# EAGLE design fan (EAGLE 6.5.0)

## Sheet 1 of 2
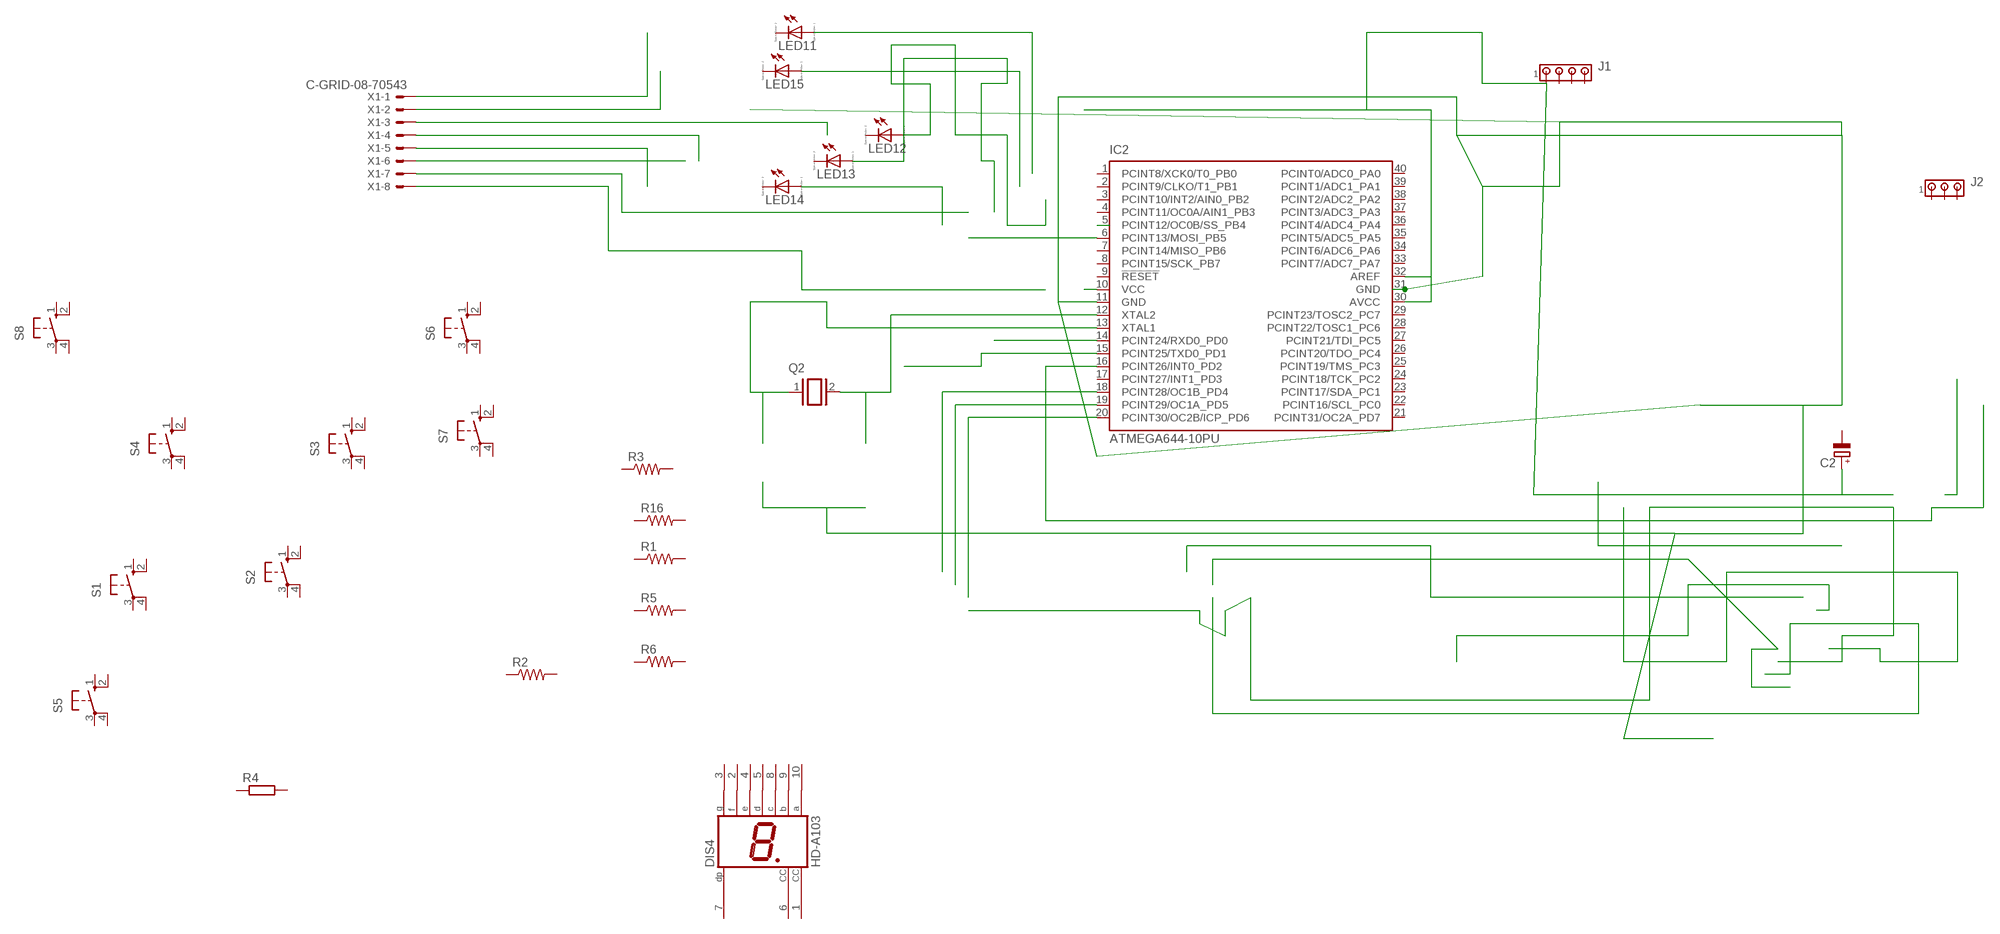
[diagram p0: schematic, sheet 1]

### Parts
C2  CPOL-EUE2,5-6E  [E2,5-6E]
DIS4  HD-A103  [HDSP-A]
IC2  ATMEGA644-10PU  [DIL40]
J1  MTA04-100  [10X04MTA]
J2  MTA03-100  [10X03MTA]
LED11  LED_ELD260  [LED_LD260]
LED12  LED_ELD260  [LED_LD260]
LED13  LED_ELD260  [LED_LD260]
LED14  LED_ELD260  [LED_LD260]
LED15  LED_ELD260  [LED_LD260]
Q2  XTAL/S  [QS]
R1  R-US_0204/2V  [0204V]
R2  R-US_0204/7  [0204/7]
R3  R-US_0204/7  [0204/7]
R4  R-EU_0207/2V  [0207/2V]
R5  R-US_0204/7  [0204/7]
R6  R-US_0204/7  [0204/7]
R16  R-US_0204/7  [0204/7]
S1  10-XX  [B3F-10XX]
S2  10-XX  [B3F-10XX]
S3  10-XX  [B3F-10XX]
S4  10-XX  [B3F-10XX]
S5  10-XX  [B3F-10XX]
S6  10-XX  [B3F-10XX]
S7  10-XX  [B3F-10XX]
S8  10-XX  [B3F-10XX]
X1  C-GRID-08-70543  [70543-08]

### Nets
N$2: IC2.13(XTAL1) Q2.1
N$3: IC2.16(PCINT26/INT0_PD2)
N$4: IC2.12(XTAL2) Q2.2
N$5: LED15.A
N$6: IC2.6(PCINT13/MOSI_PB5)
N$7: C2.+ IC2.30(AVCC) IC2.32(AREF) J1.1
N$9: LED14.A
N$11: X1.1
N$12: LED13.A
N$13: LED12.A
N$14: IC2.18(PCINT28/OC1B_PD4)
N$15: IC2.19(PCINT29/OC1A_PD5)
N$16: IC2.20(PCINT30/OC2B/ICP_PD6)
N$18: IC2.15(PCINT25/TXD0_PD1)
N$22: X1.2
N$24: X1.8
N$30: LED11.A
N$31: IC2.14(PCINT24/RXD0_PD0)
N$36: X1.4
N$37: X1.5
N$38: X1.7
N$39: X1.3
N$40: X1.6
N$43: IC2.11(GND) IC2.31(GND)
N$56: IC2.5(PCINT12/OC0B/SS_PB4)
N$66: IC2.10(VCC)
Unconnected: C2.- DIS4.1(CC) DIS4.2(F) DIS4.3(G) DIS4.4(E) DIS4.5(D) DIS4.6(CC) DIS4.7(DP) DIS4.8(C) DIS4.9(B) DIS4.10(A) IC2.1(PCINT8/XCK0/T0_PB0) IC2.2(PCINT9/CLKO/T1_PB1) IC2.3(PCINT10/INT2/AIN0_PB2) IC2.4(PCINT11/OC0A/AIN1_PB3) IC2.7(PCINT14/MISO_PB6) IC2.8(PCINT15/SCK_PB7) IC2.9(!RESET) IC2.17(PCINT27/INT1_PD3) IC2.21(PCINT31/OC2A_PD7) IC2.22(PCINT16/SCL_PC0) IC2.23(PCINT17/SDA_PC1) IC2.24(PCINT18/TCK_PC2) IC2.25(PCINT19/TMS_PC3) IC2.26(PCINT20/TDO_PC4) IC2.27(PCINT21/TDI_PC5) IC2.28(PCINT22/TOSC1_PC6) IC2.29(PCINT23/TOSC2_PC7) IC2.33(PCINT7/ADC7_PA7) IC2.34(PCINT6/ADC6_PA6) IC2.35(PCINT5/ADC5_PA5) IC2.36(PCINT4/ADC4_PA4) IC2.37(PCINT3/ADC3_PA3) IC2.38(PCINT2/ADC2_PA2) IC2.39(PCINT1/ADC1_PA1) IC2.40(PCINT0/ADC0_PA0) J1.2 J1.3 J1.4 J2.1 J2.2 J2.3 LED11.K(C) LED12.K(C) LED13.K(C) LED14.K(C) LED15.K(C) R1.1 R1.2 R2.1 R2.2 R3.1 R3.2 R4.1 R4.2 R5.1 R5.2 R6.1 R6.2 R16.1 R16.2 S1.1(S) S1.2(S1) S1.3(P) S1.4(P1) S2.1(S) S2.2(S1) S2.3(P) S2.4(P1) S3.1(S) S3.2(S1) S3.3(P) S3.4(P1) S4.1(S) S4.2(S1) S4.3(P) S4.4(P1) S5.1(S) S5.2(S1) S5.3(P) S5.4(P1) S6.1(S) S6.2(S1) S6.3(P) S6.4(P1) S7.1(S) S7.2(S1) S7.3(P) S7.4(P1) S8.1(S) S8.2(S1) S8.3(P) S8.4(P1)

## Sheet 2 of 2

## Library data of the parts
C2 = rcl:CPOL-EU: POLARIZED CAPACITOR, European symbol
DIS4 = display-hp:HD-A103: LED DISPLAY 1-character 7 segment, decimal point right; OC_FARNELL: unknown; OC_NEWARK: unknown
IC2 = atmel:ATMEGA644-*PU: 8-bit Microcontroller with 64K Bytes In-System Programmable Flash Auto generated by make-symbol-device-package-bsdl.ulp Rev. 34 Source: http://www.atmel.com/dyn/resources/prod_documents/doc2593.pdf; MPN: ATMEGA644V-10PU; OC_FARNELL: 1288342; OC_NEWARK: 23M5062
J1 = con-amp:MTA04-100: AMP connector
J2 = con-amp:MTA03-100: AMP connector
LED11-LED15 = eagle-ltspice:LED_E: LED; SPICEMODEL: NONE; SPICEPREFIX: D; SPICETYPE: diode
Q2 = special:XTAL/S: CRYSTAL
R1 = adafruit:R-US_: RESISTOR, American symbol
R2 R3 R5 R6 R16 = rcl:R-US_: RESISTOR, American symbol
R4 = rcl:R-EU_: RESISTOR, European symbol
S1-S8 = switch-omron:10-XX: OMRON SWITCH; MPN: B3F-1000; OC_FARNELL: 176432; OC_NEWARK: 36M3542
X1 = con-molex:C-GRID-08: CONNECTOR wire to board 2.54 mm (0.100") pitch header; OC_FARNELL: unknown; OC_NEWARK: unknown

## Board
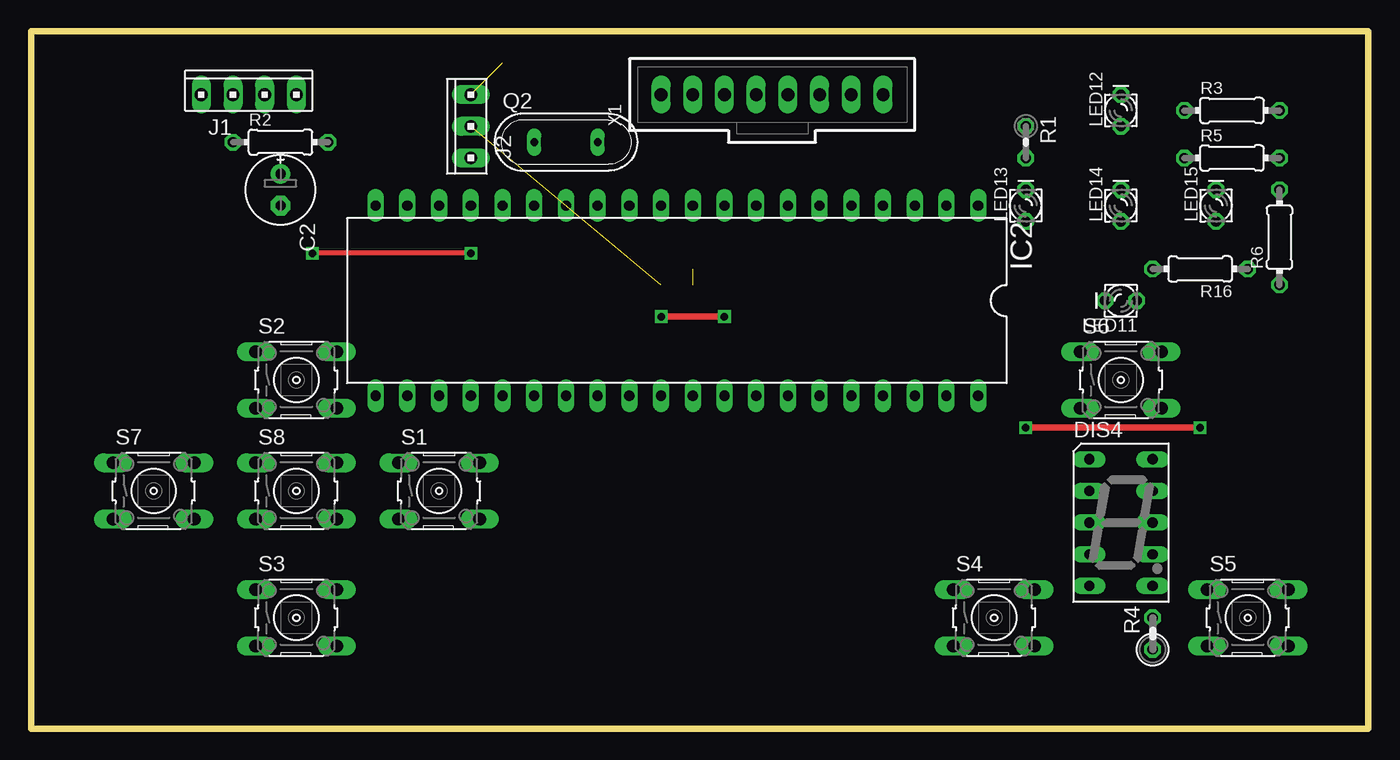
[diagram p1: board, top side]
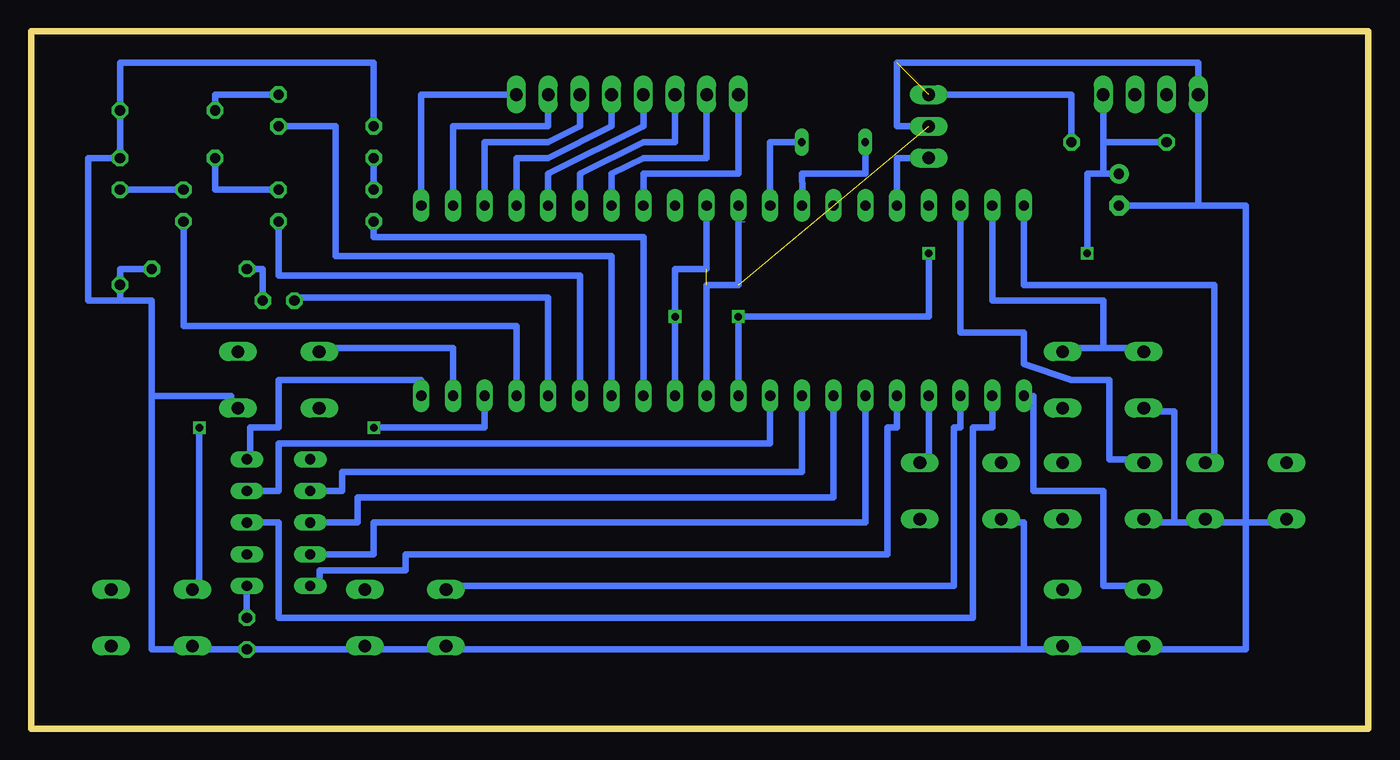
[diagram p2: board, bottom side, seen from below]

Size 107.09 x 55.88 mm. Coordinates in mm from the lower left corner, seen from the top.
Outline: 107.09,0 107.09,55.88 0,55.88 0,0 107.09,0
Copper layers (1*16): Top 0.035mm / dielectric 1.5mm / Bottom 0.035mm
Design rules "default": minimum track width 10mil, minimum drill 24mil, track to track 8mil, track to pad 8mil, pad to pad 8mil, via to via 8mil, smd to smd 8mil, copper to edge 40mil, drill to drill 8mil, minimum pad ring 10mil, minimum via ring 8mil, stop-mask expansion 4mil, vias tented up to drill 0mil, thermal gap 10mil

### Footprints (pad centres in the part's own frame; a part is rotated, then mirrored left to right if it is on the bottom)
E2,5-6E = drill 0.813 pad 1.575: + -1.27,0 | drill 0.813 pad 1.575 octagon: - 1.27,0
HDSP-A = drill 0.813 long: 1 -2.54,5.08; 2 -2.54,2.54; 3 -2.54,0; 4 -2.54,-2.54; 5 -2.54,-5.08; 6 2.54,-5.08; 7 2.54,-2.54; 8 2.54,0; 9 2.54,2.54; 10 2.54,5.08
DIL40 = drill 0.813 long: 1 -24.13,-7.62; 2 -21.59,-7.62; 3 -19.05,-7.62; 4 -16.51,-7.62; 5 -13.97,-7.62; 6 -11.43,-7.62; 7 -8.89,-7.62; 8 -6.35,-7.62; 9 -3.81,-7.62; 10 -1.27,-7.62; 11 1.27,-7.62; 12 3.81,-7.62; 13 6.35,-7.62; 14 8.89,-7.62; 15 11.43,-7.62; 16 13.97,-7.62; 17 16.51,-7.62; 18 19.05,-7.62; 19 21.59,-7.62; 20 24.13,-7.62; 21 24.13,7.62; 22 21.59,7.62; 23 19.05,7.62; 24 16.51,7.62; 25 13.97,7.62; 26 11.43,7.62; 27 8.89,7.62; 28 6.35,7.62; 29 3.81,7.62; 30 1.27,7.62; 31 -1.27,7.62; 32 -3.81,7.62; 33 -6.35,7.62; 34 -8.89,7.62; 35 -11.43,7.62; 36 -13.97,7.62; 37 -16.51,7.62; 38 -19.05,7.62; 39 -21.59,7.62; 40 -24.13,7.62
10X04MTA = drill 1.016 long: 1 3.81,0; 2 1.27,0; 3 -1.27,0; 4 -3.81,0
10X03MTA = drill 1.016 long: 1 2.54,0; 2 0,0; 3 -2.54,0
LED_LD260 = drill 0.813 octagon: A -1.27,0; K 1.27,0
QS = drill 0.61 long: 1 -2.54,0; 2 2.54,0
0204V = drill 0.813 octagon: 1 -1.27,0; 2 1.27,0
0204/7 = drill 0.813 octagon: 1 -3.81,0; 2 3.81,0
0207/2V = drill 0.813 octagon: 1 -1.27,0; 2 1.27,0
B3F-10XX = drill 1.016 long: 1 -3.251,2.261; 2 3.251,2.261; 3 -3.251,-2.261; 4 3.251,-2.261
70543-08 = drill 1.016 long: 1 -8.89,0; 2 -6.35,0; 3 -3.81,0; 4 -1.27,0; 5 1.27,0; 6 3.81,0; 7 6.35,0; 8 8.89,0

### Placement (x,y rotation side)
C2  19.96,43.18 270 top
DIS4  87.27,16.51 0 top
IC2  51.71,34.29 180 top
J1  17.42,50.8 0 top
J2  35.2,48.26 90 top
LED11  87.27,34.29 180 top
LED12  87.27,49.53 90 top
LED13  79.65,41.91 90 top
LED14  87.27,41.91 90 top
LED15  94.89,41.91 90 top
Q2  42.82,46.99 0 top
R1  79.65,46.99 270 top
R2  19.96,46.99 0 top
R3  96.16,49.53 0 top
R4  89.81,7.62 90 top
R5  96.16,45.72 0 top
R6  99.97,39.37 90 top
R16  93.62,36.83 180 top
S1  32.66,19.05 0 top
S2  21.23,27.94 0 top
S3  21.23,8.89 0 top
S4  77.11,8.89 0 top
S5  97.43,8.89 0 top
S6  87.27,27.94 0 top
S7  9.8,19.05 0 top
S8  21.23,19.05 0 top
X1  59.33,50.8 0 top

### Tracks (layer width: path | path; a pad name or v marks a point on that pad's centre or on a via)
N$1
  Bottom 0.508: 97.43,36.83 99.97,36.83 99.97,34.29
N$2
  Bottom 0: 45.36,44.45 IC2.13
  Bottom 0.508: Q2.1 40.28,44.45 45.36,44.45 45.29,41.72 45.36,41.72 IC2.13
N$3
  Bottom 0.508: 35.2,45.72 37.74,45.72 IC2.16
N$4
  Bottom 0.508: Q2.2 47.9,46.99 47.9,45.72 IC2.12 | 21.23,50.8 21.23,46.99 16.15,46.99
N$7  (via drill 0.6)
  Top 0.381: v35.2,38.1 v22.5,38.1
  Top 0.508: v50.44,33.02 v55.52,33.02
  Bottom 0.508: J1.1 21.23,44.45 | IC2.32 v55.52,33.02 | v35.2,38.1 35.2,33.02 v50.44,33.02 IC2.30 | v22.5,38.1 22.5,44.45 21.23,44.45 | 21.23,44.45 C2.+ | 92.35,45.72 92.35,43.18 87.27,43.18
N$14
  Bottom 0.508: IC2.18 32.66,35.35
N$19  (via drill 0.6)
  Top 0.508: v79.65,24.13 v93.62,24.13
  Bottom 0.005: 50.44,40.64 49.92,40.64
  Bottom 0.508: 68.22,26.67 68.22,32.26 94.89,32.26 94.89,40.64 | 27.58,6.35 97.43,6.35 97.43,26.67 | 97.43,26.67 97.43,34.29 102.51,34.29 102.51,45.72 99.97,45.72 99.97,53.34 79.65,53.34 79.65,48.26 | 63.14,26.67 63.14,36.32 87.27,36.32 87.27,40.64 | 65.68,26.67 65.68,34.54 86,34.54 86,34.29 | 87.27,48.26 82.7,48.26 82.7,37.85 60.6,37.85 60.6,26.67 | 79.65,43.18 79.65,45.72 | 19.96,41.91 13.61,41.91 | 13.61,41.91 9.8,41.91 | 12.34,21.59 12.34,35.56 27.58,35.56 27.58,41.91 | 30.12,41.91 30.12,34.29 21.23,34.29 21.23,30.48 | 21.23,30.48 17.42,30.48 | 32.66,35.56 32.66,31.75 27.58,31.75 27.58,29.21 23.77,27.94 20.73,27.94 20.73,21.59 17.42,21.59 | 35.2,21.59 35.2,26.67 | 27.58,26.67 26.82,26.67 26.82,19.05 21.23,19.05 21.23,11.43 17.42,11.43 | 15.52,16.51 5.99,16.51 | 79.65,40.64 79.65,39.37 58.06,39.37 58.06,26.67 | 32.66,26.67 32.66,24.13 33.17,24.13 33.17,11.43 74.57,11.43 | 89.81,11.43 89.81,8.89 | 40.28,26.67 40.28,16.51 79.65,16.51 79.65,13.97 84.73,13.97 | 58.06,41.91 58.06,44.45 50.44,44.45 50.44,50.8 | 45.36,26.67 45.36,20.57 82.19,20.57 82.19,19.05 84.73,19.05 | 42.82,26.67 42.82,18.54 80.92,18.54 80.92,16.51 84.73,16.51 | 60.6,41.91 60.6,44.45 58.06,45.72 52.98,45.72 52.98,50.8 | 63.14,41.91 63.14,44.45 58.06,46.99 55.52,46.99 55.52,50.8 | 65.68,41.91 65.68,44.45 58.06,48.26 58.06,50.8 | 68.22,41.91 68.22,45.72 65.68,45.72 60.6,48.26 60.6,50.8 | 70.76,41.91 70.76,46.99 65.68,46.99 63.14,48.26 63.14,50.8 | 73.3,41.91 73.3,48.26 65.68,48.26 65.68,50.8 | 15.52,16.51 15.52,25.4 17.42,25.4 | 19.96,6.35 27.58,6.35 | 27.58,6.35 27.58,16.51 28.85,16.51 | 83.46,30.48 73.3,30.48 73.3,26.67
  Bottom 0.508: 84.73,11.43 83.97,11.43 83.97,12.7 77.11,12.7 77.11,13.97 38.51,13.97 38.51,24.13 37.74,24.13 37.74,26.67 | 97.43,26.67 91.08,26.67 91.08,25.4 | 89.81,16.51 87.27,16.51 87.27,8.89 31.65,8.89 31.65,24.13 30.12,24.13 30.12,26.67 | 47.9,26.67 47.9,22.86 87.27,22.86 87.27,19.05 89.81,19.05 | 75.84,26.67 75.84,27.94 87.27,27.94 87.27,24.13 89.56,24.13 89.56,21.59 89.81,21.59 | 70.76,26.67 70.76,24.13 v79.65,24.13 | v93.62,24.13 93.62,11.43 94.89,11.43 | 15.52,16.51 17.42,16.51 | 21.23,30.48 25.04,30.48 | 75.84,41.91 75.84,50.8 68.22,50.8 | 88.54,34.29 88.54,36.83 89.81,36.83 | 87.27,50.8 92.35,50.8 92.35,49.53 | 99.97,43.18 94.89,43.18 | 13.61,53.34 13.61,41.91
N$43  (3 unrouted)
  Bottom 0: IC2.31 53.49,26.67
  Bottom 0.508: IC2.31 52.98,35.56 50.44,35.56 IC2.11 | 35.2,48.26 37.74,48.26 37.74,53.34 13.61,53.34 | 55.52,26.67 55.52,36.83 52.98,36.83 52.98,41.91 | 35.2,50.8 23.77,50.8 23.77,46.99
N$55
  Bottom 0.508: 9.8,41.91 9.8,6.35 20.49,6.35
N$59
  Bottom 0.508: 50.44,35.56 50.44,39.37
